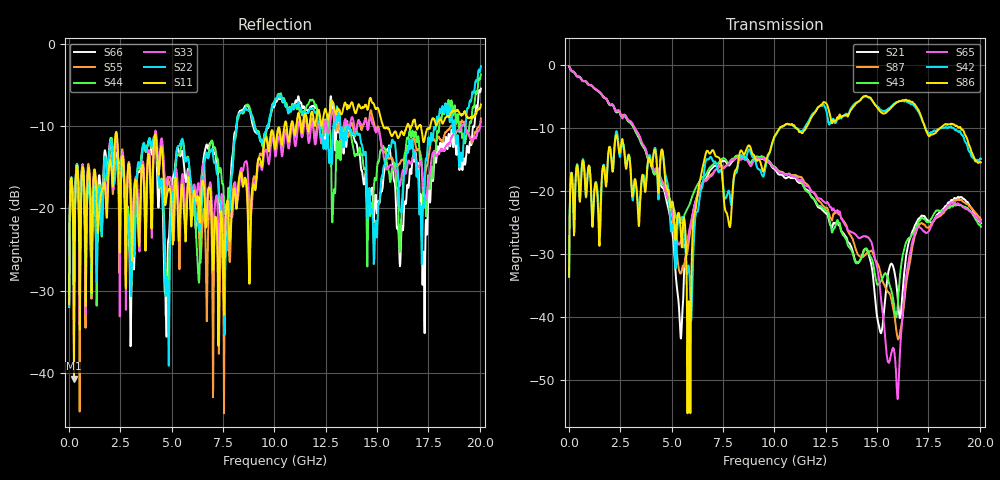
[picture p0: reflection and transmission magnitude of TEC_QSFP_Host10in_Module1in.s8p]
!!  This file represents Tyco Electronics parts only.  Due to internal design and materials, it should not  !!
!!  be used for products manufactured by companies other than Tyco Electronics.  !!
!! FILE NAME: TEC_QSFP_Host10in_Module1in.s8p
!! PART DESCRIPTION: Tyco Electronics QSFP P/N 1761987-9
!! PCB DESCRIPTION: Host Board FR4 with 10 inch microstrip, Module Board FR4 with 1.5 inch microstrip
!! FILE DESCRIPTION: 8 Port, S-Parameter, Measured Channel
!! FILE REVISION: Revision 1, 3/11/2008
!! FILE FREQUENCY RANGE: DC to 20.05 GHz in 12.50 MHz frequency steps
!! PORT DEFINITIONS:
!! Port  1  ----->  Host	Pin 24, RX4-	Module  <-----  Port  2
!! Port  3  ----->  Host	Pin 25, RX4+	Module  <-----  Port  4
!! Port  5  ----->  Host	Pin 33, TX3+	Module  <-----  Port  6
!! Port  7  ----->  Host	Pin 34, TX3-	Module  <-----  Port  8
# HZ S MA R 50.00
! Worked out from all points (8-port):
!   1604 points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, 12.5 MHz to 20.05 GHz, reference 50 ohm
!   strongest paths, dB at 12.5 MHz, 5.025 GHz, 10.04 GHz, 15.05 GHz, 20.05 GHz:
!     S86: -33.6, -21.7, -11.1, -7.0, -15.5
!     S42: -33.6, -25.7, -11.3, -6.7, -14.9
!     S65: -0.2, -23.2, -16.3, -32.9, -25.0
!     S43: -0.2, -22.1, -16.2, -34.8, -25.7
!     S87: -0.2, -23.9, -16.2, -31.7, -24.5
!     S21: -0.2, -26.3, -16.6, -40.8, -25.1
!   lowest |S11| = -40.7 dB at 250 MHz (marker M1), VSWR 1.02, Z = 50.9 + j0.0338 ohm
!   |S11| at or under -10 dB: start of sweep to 10.49 GHz; 15.3 GHz to 16.45 GHz (1.152 GHz wide, 7.25 % of centre); 17.13 GHz to 17.59 GHz (454.9 MHz wide, 2.62 % of centre)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
